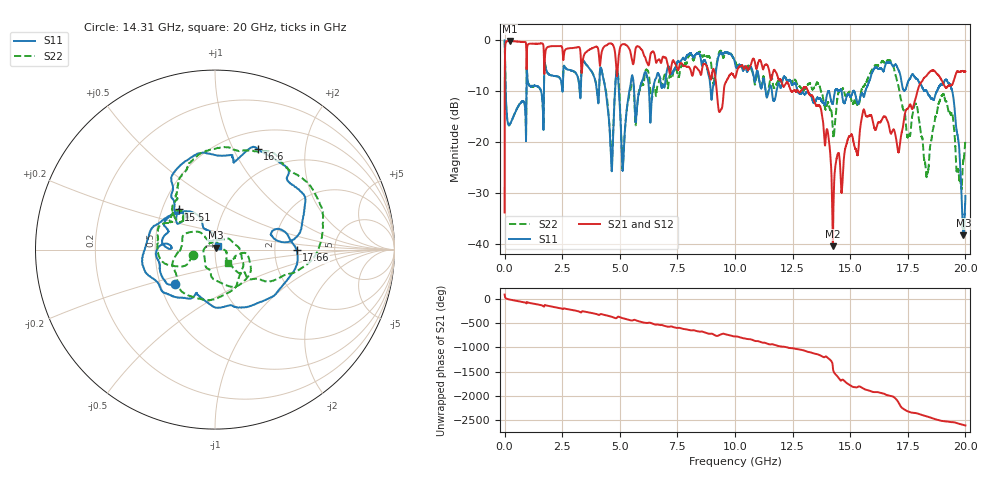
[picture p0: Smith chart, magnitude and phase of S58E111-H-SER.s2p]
!{S58E111}
!Johanson Technology Inc.
!www.johansontechnology.com
!Test Board Conditions:
!Substrate Type  RO4350B
!Substrate Thickness  60 mil
!Substrate Dk  3.66
!TL Type: GCPW
!TL Trace Width  115 mil
!TL Gap  52 mil
!Electrode orientation  Horizontal
!DUT TOPOLOGY	SERIES
!Mounting Pad LxW  55x428 mil
! Created Wed Apr 14 11:02:04 2021
# mhz S ma R 50
! 2 Port Network Data from SP1.SP block
! freq  magS11  angS11  magS21  angS21  magS12  angS12  magS22  angS22
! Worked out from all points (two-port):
!   20001 points, 300 kHz to 20 GHz, reference 50 ohm
!   highest |S21| = -0.10 dB at 227.3 MHz (marker M1); lowest = -40.4 dB at 14.25 GHz (marker M2)
!   |S21| within 3 dB of the highest: 14.52 MHz to 947.9 MHz (933.4 MHz wide, 194 % of centre); 1.755 GHz to 2.532 GHz (777 MHz wide, 36.3 % of centre)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
!   lowest |S11| = -38.2 dB at 19.92 GHz (marker M3), VSWR 1.02, Z = 50.5 + j1.12 ohm
!   |S11| at or under -10 dB: 46.47 MHz to 948.8 MHz (902.3 MHz wide, 181 % of centre); 12.73 GHz to 14.05 GHz (1.319 GHz wide, 9.85 % of centre); 19.43 GHz to end of sweep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
!   |S22| runs from -29.2 to 0.0 dB; largest |S21 - S12| = 0.011
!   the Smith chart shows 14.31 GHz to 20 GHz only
!   S11 on the Smith chart (normalised r, x): 14.31 GHz: 0.60, -0.25; 15.51 GHz: 0.61, +0.30; 16.6 GHz: 0.70, +1.25; 17.66 GHz: 2.67, -0.02; 20 GHz: 1.04, +0.05
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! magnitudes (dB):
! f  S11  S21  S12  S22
! 300 kHz  0.0  -33.8  -33.8  0.0
! 103.3 MHz  -15.0  -0.2  -0.2  -15.0
! 227.3 MHz  -16.4  -0.1  -0.1  -16.4
! 3.334 GHz  -5.6  -6.1  -6.1  -5.5
! 4.233 GHz  -6.3  -2.0  -2.0  -6.3
! 4.632 GHz  -24.5  -0.6  -0.6  -23.2
! 4.893 GHz  -5.8  -6.7  -6.7  -5.7
! 5.14 GHz  -24.8  -0.7  -0.7  -24.3
! 5.499 GHz  -7.6  -3.2  -3.2  -8.6
! 6.667 GHz  -6.5  -3.8  -3.9  -8.4
! 10 GHz  -4.5  -7.3  -7.3  -4.1
! 13.33 GHz  -11.3  -10.7  -10.8  -9.4
! 14.25 GHz  -12.4  -40.4  -39.1  -17.5
! 14.31 GHz  -10.7  -27.3  -27.3  -18.0
! 15.51 GHz  -10.4  -15.1  -15.0  -9.5
! 16.6 GHz  -4.3  -15.6  -15.6  -4.0
! 16.67 GHz  -4.4  -16.4  -16.6  -3.9
! 17.66 GHz  -6.8  -13.3  -13.3  -15.7
! 18.33 GHz  -10.0  -6.9  -6.9  -26.7
! 19.37 GHz  -9.0  -8.8  -8.7  -14.6
! 19.92 GHz  -38.2  -6.1  -6.0  -23.6
! 20 GHz  -30.5  -6.1  -6.0  -19.6
